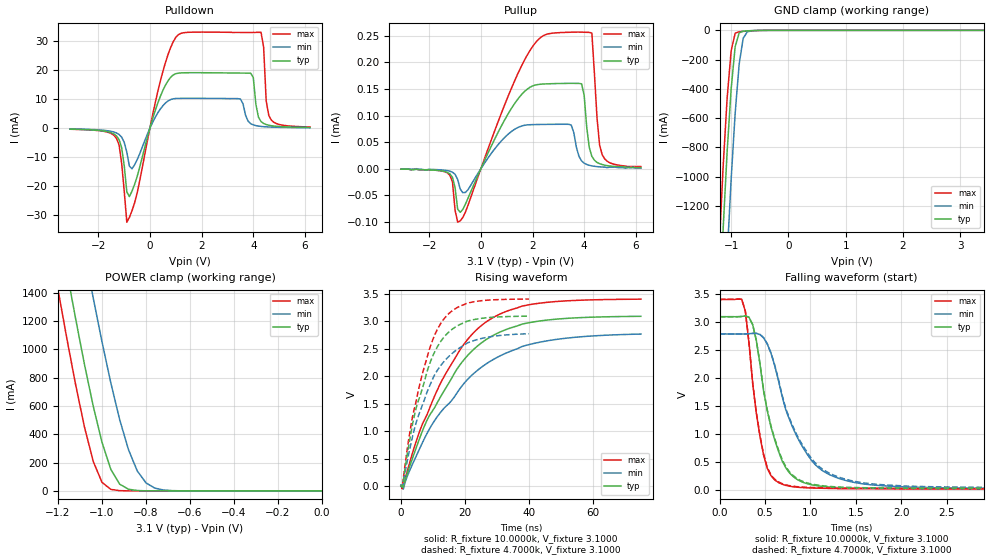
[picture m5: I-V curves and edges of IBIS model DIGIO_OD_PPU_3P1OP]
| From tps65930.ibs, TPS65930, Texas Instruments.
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|   Model DIGIO_OD_PPU_3P1OP
[Model]   DIGIO_OD_PPU_3P1OP
Model_type   I/O
Polarity   Non-Inverting
Enable   Active-Low
Vinl =   1.1935V
Vinh =   1.8135V
Vmeas =   1.6500V
Cref =  30.0000pF
Rref = 100.0000M
Vref =  0.000V
C_comp   1.0815pF   1.5672pF   1.3441pF
[Temperature Range]   25.0000   0.1250k   -40.0000
[Pullup Reference]   3.1000V   2.7900V   3.4100V
[Pulldown Reference]   0.000V   0.000V   0.000V
[POWER Clamp Reference]   3.1000V   2.7900V   3.4100V
[GND Clamp Reference]   0.000V   0.000V   0.000V
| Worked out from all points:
|   slope of the pulldown table from 0 to 0.465 V, typ, clamps not added: 38.3 ohm
|   GND clamp passes 1 mA (typ) near -0.54 V on its own axis
|   POWER clamp passes 1 mA (typ) near -0.81 V on its own axis
|   rising waveform, R_fixture 10.0000k, V_fixture 3.1000: 20-80 % time 18.1ns typ, 21.5ns min, 17.6ns max; typ from 0.01 V to 3.09 V
|   rising waveform, R_fixture 4.7000k, V_fixture 3.1000: 20-80 % time 8.71ns typ, 10.4ns min, 8.36ns max; typ from 0.021 V to 3.1 V
|   falling waveform, R_fixture 10.0000k, V_fixture 3.1000: 20-80 % time 239ps typ, 386ps min, 160ps max; typ from 3.1 V to 0.012 V
|   falling waveform, R_fixture 4.7000k, V_fixture 3.1000: 20-80 % time 242ps typ, 394ps min, 161ps max; typ from 3.1 V to 0.024 V
[Pulldown]
| voltage   I(typ)   I(min)   I(max)
-3.1V     -362uA     -294uA     -377uA
-1.3V     -2.689mA   -1.667mA   -3.506mA
-1.1V     -6.692mA   -3.096mA   -12.07mA
-900mV    -21.92mA   -8.254mA   -32.33mA
-700mV    -21.68mA   -13.98mA   -28.43mA
700mV     16.32mA    9.359mA    25.36mA
1.8V      19.05mA    10.24mA    33mA
3.5V      18.92mA    10.02mA    32.9mA
3.9V      18.88mA    1.529mA    32.88mA
4.3V      2.265mA    589.4uA    32.91mA
4.6V      990.3uA    397.5uA    4.368mA
6.2V      237uA      143uA      391uA
[Pullup]
| voltage   I(typ)   I(min)   I(max)
-3.1V     -1uA       -1uA       -1uA
-1.3V     -6.9uA     -3.6uA     -7.9uA
-800mV    -81.99uA   -38.27uA   -98.03uA
900mV     89.88uA    57.72uA    117.5uA
1.9V      153.1uA    82.69uA    222.1uA
3.5V      160.5uA    82.18uA    256.7uA
3.7V      160.4uA    40.26uA    256.9uA
4V        138.5uA    10.4uA     256.6uA
4.3V      23.2uA     5.3uA      254.9uA
4.5V      11.8uA     3.9uA      95.04uA
4.7V      7.8uA      3.1uA      26.3uA
6.2V      2uA        1uA        4uA
[GND_clamp]
| voltage   I(typ)   I(min)   I(max)
-3.1V     -20.18A    -20.88A    -19.81A
-1.21V    -1.944A    -2.722A    -1.496A
-1.14V    -1.358A    -2.119A    -931.7mA
-1.07V    -828.2mA   -1.545A    -463.2mA
-1V       -400.1mA   -1.017A    -139.5mA
-930mV    -111.5mA   -566.8mA   -19.63mA
-860mV    -17.2mA    -230.7mA   -9.756mA
-790mV    -5.711mA   -54.5mA    -7.195mA
-720mV    -3.473mA   -10.96mA   -5.135mA
-650mV    -2.254mA   -3.258mA   -3.378mA
-440mV    -340.6uA   -330.5uA   -480.4uA
3.41V     0A         0A         0A
[POWER_clamp]
| voltage   I(typ)   I(min)   I(max)
-3.08V    20.1A      20.83A     19.69A
-1.2V     1.902A     2.726A     1.422A
-1.16V    1.554A     2.374A     1.078A
-1.12V    1.217A     2.028A     750.9mA
-1.04V    599.1mA    1.364A     208.6mA
-1V       342.7mA    1.053A     60.09mA
-960mV    152mA      763.2mA    10.89mA
-920mV    48.17mA    505mA      1.914mA
-840mV    2.737mA    141.5mA    328.4uA
-800mV    698.6uA    56.57mA    251.6uA
-680mV    95.12uA    2.068mA    134.3uA
0V        82.52pA    3.215nA    53.13pA
[Ramp]
| variable   typ   min   max
dV/dt_r   3.0995n/5.504e-17  10.7287n/0.2054n  5.6915n/2.151e-17
|dV/dt_r   n/-2.151e-17
dV/dt_f   0.5682/0.3355n   0.3056/0.4031n   0.9840/0.3001n
R_load = 50.0000
[Rising Waveform]
R_fixture = 10.0000k
V_fixture = 3.1000
V_fixture_min = 2.7900
V_fixture_max = 3.4100
| time   V(typ)   V(min)   V(max)
0s        9.833mV    14.04mV    7.664mV
757.6ps   -16.2mV    -56.47mV   7.053mV
4.546ns   656.9mV    514.2mV    773.9mV
7.576ns   1.122V     891.1mV    1.228V
12.88ns   1.674V     1.377V     1.928V
18.94ns   2.245V     1.813V     2.521V
25.76ns   2.633V     2.189V     2.952V
33.33ns   2.861V     2.434V     3.191V
43.18ns   3.006V     2.619V     3.331V
75ns      3.093V     2.769V     3.405V
[Rising Waveform]
R_fixture = 4.7000k
V_fixture = 3.1000
V_fixture_min = 2.7900
V_fixture_max = 3.4100
| time   V(typ)   V(min)   V(max)
0s        20.92mV    29.91mV    16.3mV
404ps     -22.96mV   292.6uV    -50.86mV
808.1ps   118.2mV    35mV       157.1mV
3.232ns   997.5mV    793.7mV    1.13V
6.465ns   1.73V      1.436V     1.986V
9.293ns   2.275V     1.867V     2.558V
12.93ns   2.673V     2.231V     3.003V
16.97ns   2.895V     2.461V     3.23V
22.22ns   3.025V     2.639V     3.351V
40ns      3.095V     2.775V     3.407V
[Falling Waveform]
R_fixture = 10.0000k
V_fixture = 3.1000
V_fixture_min = 2.7900
V_fixture_max = 3.4100
| time   V(typ)   V(min)   V(max)
0s        3.1V       2.79V      3.41V
242.4ps   3.105V     2.79V      3.413V
282.8ps   3.114V     2.791V     3.197V
363.6ps   2.956V     2.801V     1.901V
484.8ps   1.756V     2.72V      608.1mV
646.5ps   692.3mV    1.961V     127.7mV
727.3ps   392.4mV    1.434V     76mV
929.3ps   123.2mV    723.5mV    34.2mV
1.293ns   36.41mV    211.7mV    17.8mV
4ns       12.36mV    18.63mV    7.68mV
[Falling Waveform]
R_fixture = 4.7000k
V_fixture = 3.1000
V_fixture_min = 2.7900
V_fixture_max = 3.4100
| time   V(typ)   V(min)   V(max)
0s        3.1V       2.79V      3.41V
242.4ps   3.105V     2.79V      3.413V
282.8ps   3.114V     2.791V     3.198V
363.6ps   2.957V     2.801V     1.911V
484.8ps   1.772V     2.72V      626.5mV
646.5ps   716.1mV    1.979V     138.8mV
727.3ps   413.8mV    1.456V     85.81mV
888.9ps   165.6mV    863.3mV    47.17mV
1.293ns   48.17mV    235.5mV    26.53mV
4ns       23.56mV    34.47mV    16.31mV
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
